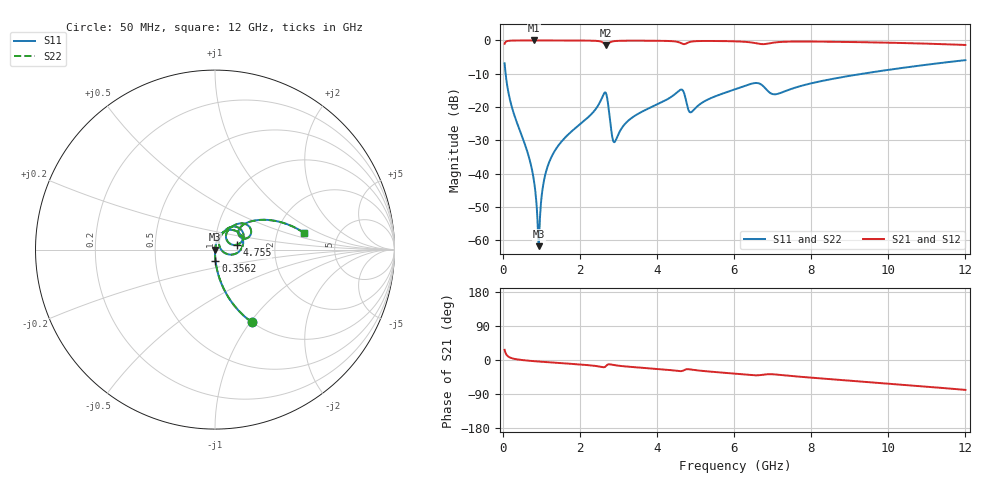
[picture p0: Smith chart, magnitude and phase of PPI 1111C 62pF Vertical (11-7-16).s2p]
# GHz S MA R 50
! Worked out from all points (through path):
!   1601 points, 50 MHz to 12 GHz, reference 50 ohm
!   highest |S21| = -0.01 dB at 819.3 MHz (marker M1); lowest = -1.4 dB at 2.686 GHz (marker M2)
!   group delay of S21, straight-line fit = 18.3 ps
!   lowest |S11| = -61.7 dB at 931.3 MHz (marker M3), VSWR 1.00, Z = 50.1 - j0.0134 ohm
!   |S11| at or under -10 dB: 76.26 MHz to 9.329 GHz (9.252 GHz wide, 197 % of centre)
!   |S22| runs from -61.7 to -5.9 dB; largest |S21 - S12| = 0
!   S11 on the Smith chart (normalised r, x): 50 MHz: 1.00, -1.02; 356.2 MHz: 1.00, -0.12; 4.755 GHz: 1.27, +0.07; 12 GHz: 2.86, +0.70
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0.05  0.4542 -63.2  0.8906 26.8  0.8906 26.8  0.4542 -63.2
0.3562187  0.06138 -87.5  0.9976 2.0  0.9976 2.0  0.06138 -87.5
0.6699063  0.01871 -89.7  0.9991 -1.8  0.9991 -1.8  0.01871 -89.7
0.8192812  0.007297 -87.1  0.9992 -3.1  0.9992 -3.1  0.007297 -87.1
0.9313125  0.0008201 -9.4  0.9991 -4.0  0.9991 -4.0  0.0008201 -9.4
1.073219  0.008041 78.6  0.999 -5.1  0.999 -5.1  0.008041 78.6
1.237531  0.0165 80.4  0.9988 -6.3  0.9988 -6.3  0.0165 80.4
2.044156  0.05771 75.7  0.9961 -12.2  0.9961 -12.2  0.05771 75.7
2.686469  0.157 8.7  0.8543 -15.3  0.8543 -15.3  0.157 8.7
2.835844  0.03749 -6.4  0.9625 -12.5  0.9625 -12.5  0.03749 -6.4
2.903062  0.02994 29.0  0.9776 -13.7  0.9776 -13.7  0.02994 29.0
3.283969  0.06456 66.9  0.9918 -17.8  0.9918 -17.8  0.06456 66.9
4.038312  0.1118 63.5  0.9881 -23.7  0.9881 -23.7  0.1118 63.5
4.613406  0.1823 39.2  0.9192 -29.5  0.9192 -29.5  0.1823 39.2
4.755312  0.1247 12.6  0.8976 -24.7  0.8976 -24.7  0.1247 12.6
4.88975  0.08404 38.1  0.9592 -25.2  0.9592 -25.2  0.08404 38.1
6.025  0.1848 49.7  0.9691 -36.2  0.9691 -36.2  0.1848 49.7
6.600094  0.2297 30.5  0.9009 -40.4  0.9009 -40.4  0.2297 30.5
7.070625  0.1557 31.2  0.934 -38.2  0.934 -38.2  0.1557 31.2
8.019156  0.2285 40.3  0.9614 -46.7  0.9614 -46.7  0.2285 40.3
10.01331  0.3627 26.5  0.9247 -62.4  0.9247 -62.4  0.3627 26.5
12  0.5065 10.4  0.855 -78.9  0.855 -78.9  0.5065 10.4
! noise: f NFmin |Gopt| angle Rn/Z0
0.05  0.0003537  0.8598  0.552  0.00054
1.372  0.003694  0.6695  5.842  0.002143
2.701  0.06386  0.9561  11.66  0.3245
4.031  0.01422  0.7411  17.01  0.01077
5.36  0.02138  0.7702  22.57  0.01826
6.682  0.07937  0.9177  28.17  0.2004
8.012  0.02951  0.7612  32.99  0.02307
9.341  0.02498  0.6917  37.3  0.01422
10.67  0.02571  0.6712  41.51  0.01323
12  0.02791  0.6702  45.64  0.01392
